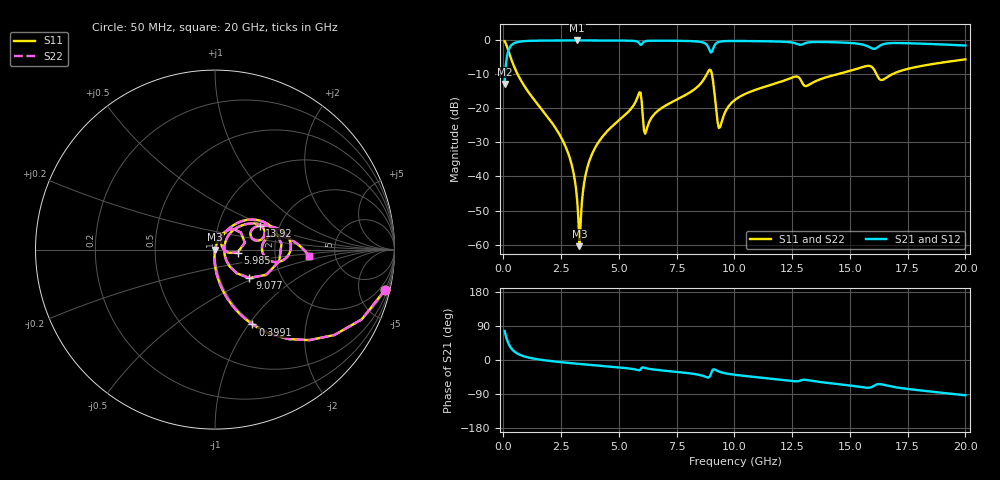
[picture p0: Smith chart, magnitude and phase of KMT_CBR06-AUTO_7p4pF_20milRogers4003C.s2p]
! Data measured by Modelithics Inc. support@modelithics.com 813-866-6335
! KEMET CBR06-AUTO 7.4pF, Pad Width= 0.851mm, Pad Length= 0.64mm, Pad Gap= 0.62mm, 20mil Rogers 4003C substrate Data, January 2022
# hz S ma R 50
! 2 Port Network Data from SP1.SP block
! freq  magS11  angS11  magS21  angS21  magS12  angS12  magS22  angS22
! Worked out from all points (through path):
!   401 points, 50 MHz to 20 GHz, reference 50 ohm
!   highest |S21| = -0.01 dB at 3.192 GHz (marker M1); lowest = -12.8 dB at 50 MHz (marker M2)
!   group delay of S21, straight-line fit = 14.2 ps
!   lowest |S11| = -60.5 dB at 3.292 GHz (marker M3), VSWR 1.00, Z = 50.1 - j0.0341 ohm
!   |S11| at or under -10 dB: 618.4 MHz to 8.798 GHz (8.179 GHz wide, 174 % of centre); 9.029 GHz to 14.42 GHz (5.391 GHz wide, 46 % of centre); 16.16 GHz to 16.82 GHz (659.6 MHz wide, 4 % of centre)
!   |S22| runs from -60.5 to -0.2 dB; largest |S21 - S12| = 0
!   S11 on the Smith chart (normalised r, x): 50 MHz: 0.98, -8.43; 399.1 MHz: 0.98, -1.04; 5.985 GHz: 1.29, -0.05; 9.077 GHz: 1.38, -0.47; 13.92 GHz: 1.58, +0.46; 20 GHz: 3.19, -0.32
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5e7  0.9735 -13.4  0.2283 76.6  0.2283 76.6  0.9735 -13.4
3.99125e8  0.466 -63.4  0.8842 26.5  0.8842 26.5  0.466 -63.4
2.6435e9  0.02977 -95.1  0.9986 -6.7  0.9986 -6.7  0.02977 -95.1
2.992625e9  0.01312 -94.9  0.9989 -8.7  0.9989 -8.7  0.01312 -94.9
3.192125e9  0.004464 -88.0  0.999 -9.9  0.999 -9.9  0.004464 -88.0
3.291875e9  0.0009455 -21.1  0.999 -10.4  0.999 -10.4  0.0009455 -21.1
3.391625e9  0.004037 65.5  0.9989 -11.0  0.9989 -11.0  0.004037 65.5
3.591125e9  0.01194 73.2  0.9988 -12.1  0.9988 -12.1  0.01194 73.2
4.04e9  0.02912 73.4  0.9984 -14.5  0.9984 -14.5  0.02912 73.4
5.8355e9  0.1564 45.7  0.942 -27.0  0.942 -27.0  0.1564 45.7
5.985125e9  0.1266 -7.9  0.8758 -20.5  0.8758 -20.5  0.1266 -7.9
6.184625e9  0.04726 43.7  0.9794 -22.0  0.9794 -22.0  0.04726 43.7
6.73325e9  0.09508 60.9  0.9912 -26.7  0.9912 -26.7  0.09508 60.9
8.678375e9  0.2686 38.6  0.9229 -42.7  0.9229 -42.7  0.2686 38.6
9.077375e9  0.2481 -39.5  0.7576 -24.9  0.7576 -24.9  0.2481 -39.5
9.376625e9  0.05299 12.7  0.961 -31.5  0.961 -31.5  0.05299 12.7
1.0025e10  0.1339 47.2  0.9821 -39.1  0.9821 -39.1  0.1339 47.2
1.336662e10  0.2371 28.7  0.9462 -55.2  0.9462 -55.2  0.2371 28.7
1.391525e10  0.2828 28.1  0.9475 -59.6  0.9475 -59.6  0.2828 28.1
1.576062e10  0.4222 4.8  0.8221 -73.1  0.8221 -73.1  0.4222 4.8
1.670825e10  0.3018 12.7  0.91 -69.0  0.91 -69.0  0.3018 12.7
2e10  0.5269 -3.9  0.8419 -93.1  0.8419 -93.1  0.5269 -3.9
